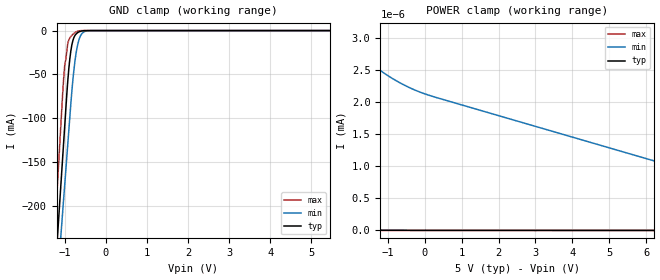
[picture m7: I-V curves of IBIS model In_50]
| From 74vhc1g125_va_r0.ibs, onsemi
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|//////////////////////////////////////////////////////////////////////////////
|//////////////////////////////////////////////////////////////////////////////
[Model]  In_50
Model_type Input
Vinh = 3.50
Vinl = 1.50
|  variable   typ   min   max
C_comp   2.7pF   2.7pF   2.7pF
|//////////////////////////////////////////////////////////////////////////////
[Temperature Range]   25   125   -55
|//////////////////////////////////////////////////////////////////////////////
[Voltage Range]   5.00V   4.50V   5.50V
|//////////////////////////////////////////////////////////////////////////////
[POWER Clamp Reference] 5.00V   4.50V   5.50V
|//////////////////////////////////////////////////////////////////////////////
[GND Clamp Reference]   0V   0V   0V
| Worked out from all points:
|   GND clamp passes 1 mA (typ) near -0.63 V on its own axis
|   POWER clamp passes 1 mA (typ) near -4.99 V on its own axis
|//////////////////////////////////////////////////////////////////////////////
[GND Clamp]
|   Voltage   I(typ)   I(min)   I(max)
-5V       -2.973A    -2.656A    -3.292A
-1.25V    -287.2mA   -330.1mA   -234.3mA
-1.175V   -233.5mA   -283.6mA   -173.2mA
-1.075V   -161.9mA   -221.6mA   -91.64mA
-1V       -108.1mA   -175.1mA   -39.14mA
-925mV    -56.43mA   -128.5mA   -13.96mA
-850mV    -22.53mA   -82.03mA   -6.643mA
-775mV    -7.602mA   -43.76mA   -3.101mA
-700mV    -2.845mA   -19.24mA   -966.2uA
-600mV    -609uA     -4.563mA   -52.45uA
-425mV    -3.575uA   -168.8uA   -18.21nA
5.45V     1.61pA     2.28nA     400.7fA
|//////////////////////////////////////////////////////////////////////////////
[POWER Clamp]
|   Voltage   I(typ)   I(min)   I(max)
-5V       1.191mA    8.677nA    31.48mA
-4.775V   3.1nA      7.537nA    26.8mA
-4.7V     2.237nA    7.22nA     25.08mA
-4.625V   1.784nA    6.931nA    23.26mA
-4.4V     994.6pA    6.187nA    17.03mA
-4.175V   595.4pA    5.583nA    9.534mA
-3.8V     272.9pA    4.796nA    6.926uA
-3.725V   231.2pA    4.666nA    8.566pA
-2.3V     15.55pA    3.105nA    536.9fA
-1.325V   4.701pA    2.543nA    475.1fA
-125mV    1.733pA    2.153nA    410.1fA
10V       -315.6fA   448.2pA    -137.9fA
